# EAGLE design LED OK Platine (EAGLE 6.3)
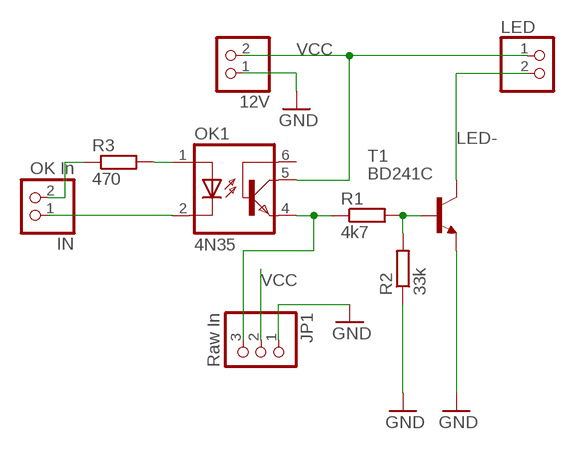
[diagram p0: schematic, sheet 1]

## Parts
12V  PINHD-1X02_2.54-90°  [1X02/90]
IN  OK In  PINHD-1X02_2.54-90°  [1X02/90]
JP1  Raw In  PINHD-1X03_2.54-90°  [1X03/90]
LED  PINHD-1X02_2.54-90°  [1X02/90]
OK1  4N35  [DIL06]
R1  4k7  R-EU_0207/10  [0207/10]
R2  33k  R-EU_0207/10  [0207/10]
R3  470  R-EU_0207/2V  [0207/2V]
T1  BD241C  2N5496  [TO220]

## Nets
GND: 12V.1 JP1.1 R2.1 T1.3(E)
LED-: LED.2 T1.2(C)
N$1: IN.2 R3.1
N$2: IN.1 OK1.2(C)
N$3: OK1.1(A) R3.2
N$4: JP1.3 OK1.4(EMI) R1.1
N$5: R1.2 R2.2 T1.1(B)
VCC: 12V.2 JP1.2 LED.1 OK1.5(COL)
Unconnected: OK1.6(BAS)

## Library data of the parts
12V IN LED = pinhead-2:PINHD-1X02: PIN HEADER
JP1 = pinhead-2:PINHD-1X03: PIN HEADER
OK1 = optocoupler:4N35: MOTOROLA OPTO COUPLER; MF: FAIRCHILD SEMICONDUCTOR; MPN: 4N35; OC_FARNELL: 1328375; OC_NEWARK: 72K9946
R1-R3 = resistor:R-EU_: RESISTOR, European symbol
T1 = transistor:2N5496: NPN TRANSISTOR

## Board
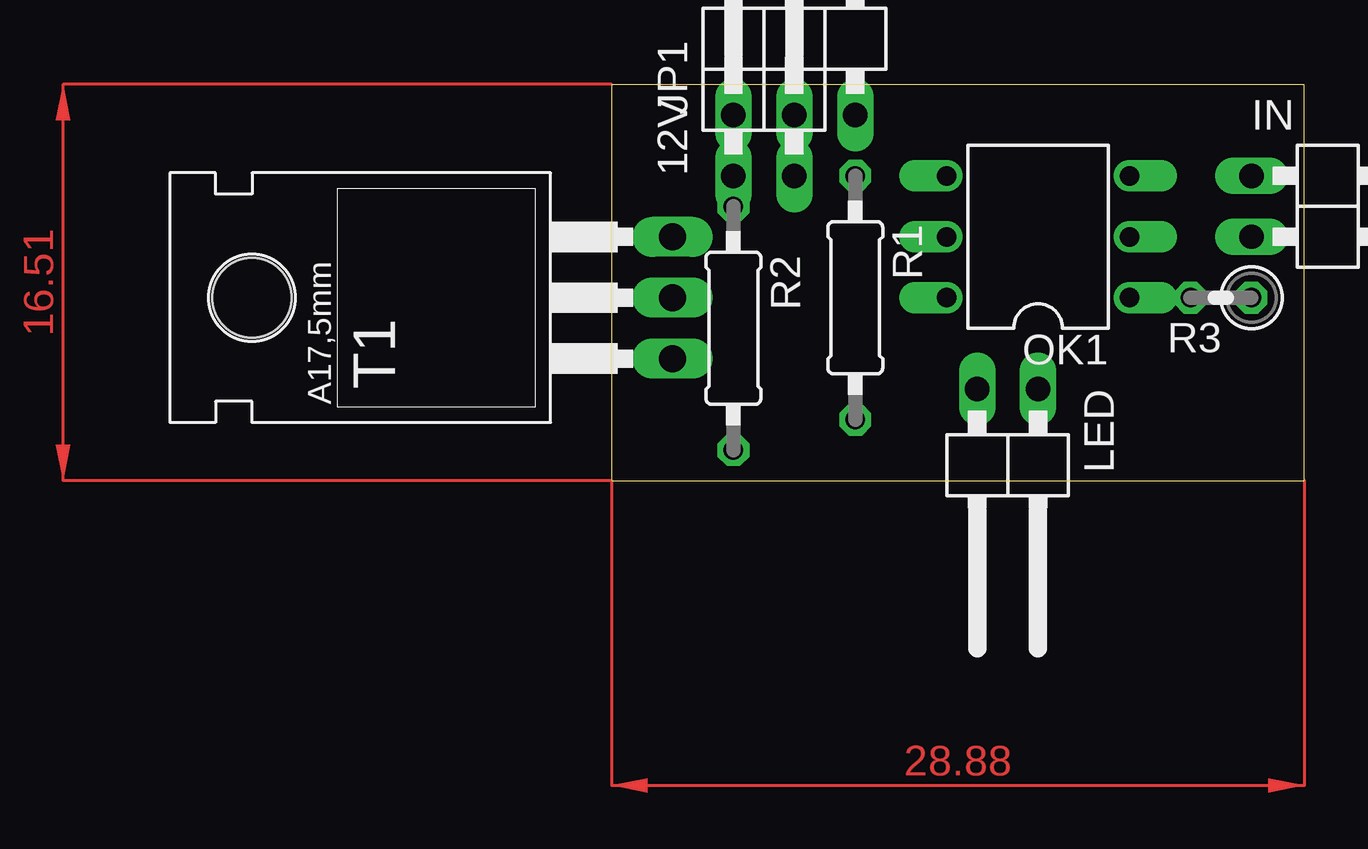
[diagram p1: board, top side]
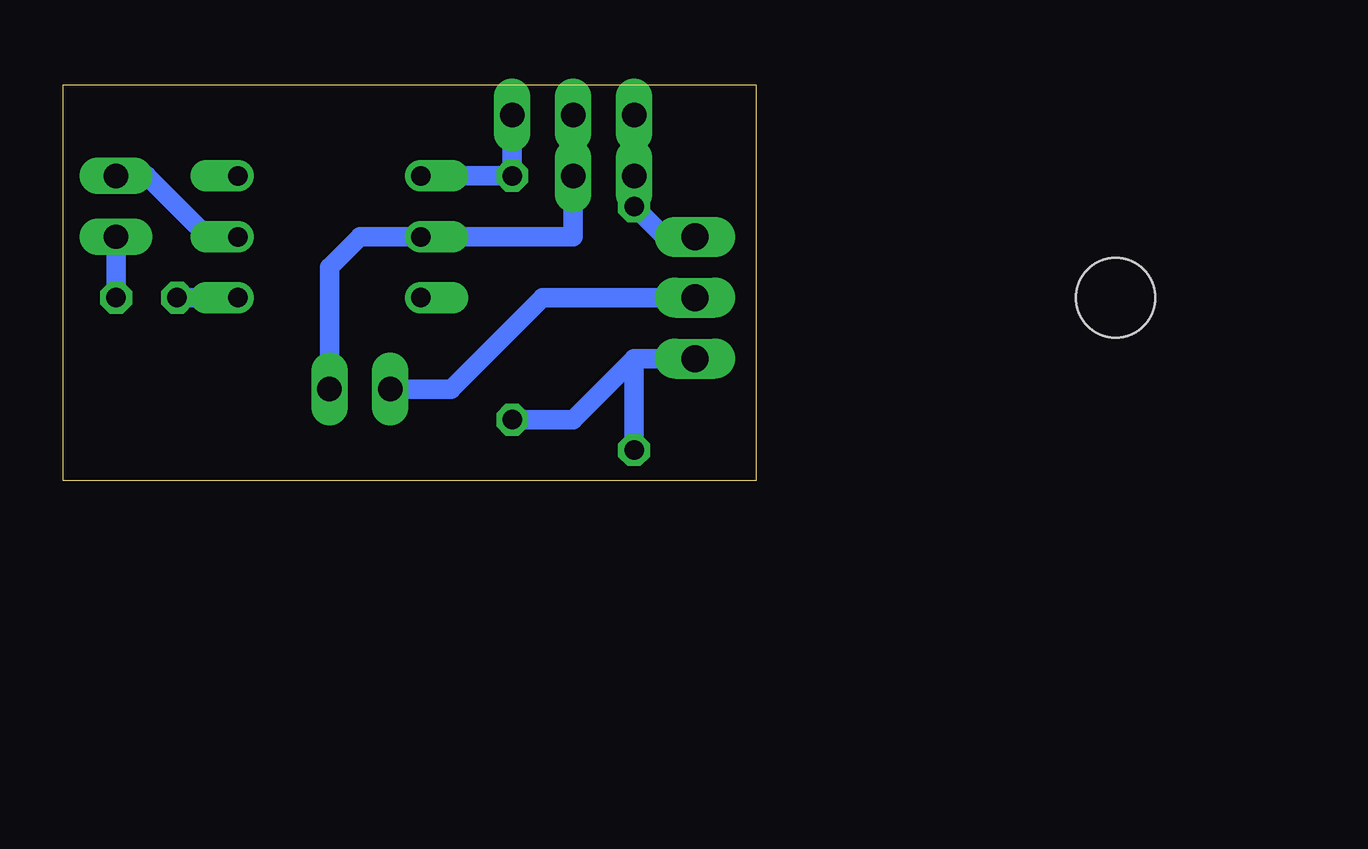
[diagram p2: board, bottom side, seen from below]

Size 28.88 x 16.5 mm. Coordinates in mm from the lower left corner, seen from the top.
Outline: 0,0 28.88,0 28.88,16.5 0,16.5 0,0
Copper layers (1*16): Top 0.035mm / dielectric 1.5mm / Bottom 0.035mm
Design rules "default": minimum track width 10mil, minimum drill 24mil, track to track 8mil, track to pad 8mil, pad to pad 8mil, via to via 8mil, smd to smd 8mil, copper to edge 40mil, drill to drill 8mil, minimum pad ring 10mil, minimum via ring 8mil, stop-mask expansion 4mil, vias tented up to drill 0mil, thermal gap 10mil

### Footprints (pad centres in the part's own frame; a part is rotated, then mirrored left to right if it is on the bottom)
1X02/90 = drill 1.016 long: 1 -2.54,-3.81; 2 0,-3.81
1X03/90 = drill 1.016 long: 1 -2.54,-3.81; 2 0,-3.81; 3 2.54,-3.81
DIL06 = drill 0.813 offset: 1 -2.54,-3.81; 2 0,-3.81; 3 2.54,-3.81; 4 2.54,3.81; 5 0,3.81; 6 -2.54,3.81
0207/10 = drill 0.813 octagon: 1 -5.08,0; 2 5.08,0
0207/2V = drill 0.813 octagon: 1 -1.27,0; 2 1.27,0
TO220 = drill 1.118 long: 1 -2.54,-6.35; 2 0,-6.35; 3 2.54,-6.35 | hole 3.302: 0,11.176

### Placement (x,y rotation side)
12V  7.62,16.51 0 top
IN  30.48,10.16 270 top
JP1  7.62,19.05 0 top
LED  15.24,0 180 top
OK1  17.78,10.16 90 top
R1  10.16,7.62 270 top
R2  5.08,6.35 270 top
R3  25.4,7.62 180 top
T1  -3.81,7.62 90 top

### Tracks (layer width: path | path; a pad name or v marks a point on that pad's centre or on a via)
GND
  Bottom 0.813: T1.3 3.81,10.16 R2.1 12V.1 JP1.1
LED-
  Bottom 0.813: T1.2 8.89,7.62 12.7,3.81 LED.2
N$1
  Bottom 0.813: IN.2 R3.1
N$2
  Bottom 0.813: OK1.2 22.86,10.16 25.4,12.7 IN.1
N$3
  Bottom 0.813: R3.2 OK1.1
N$4
  Bottom 0.813: OK1.4 R1.1 JP1.3
N$5
  Bottom 0.813: T1.1 5.08,5.08 | 5.08,5.08 7.62,2.54 R1.2 | R2.2 5.08,5.08
VCC
  Bottom 0.813: LED.1 17.78,8.89 16.51,10.16 OK1.5 7.62,10.16 12V.2 JP1.2
(copper drawn outside any net)
  shapes: Top area x2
